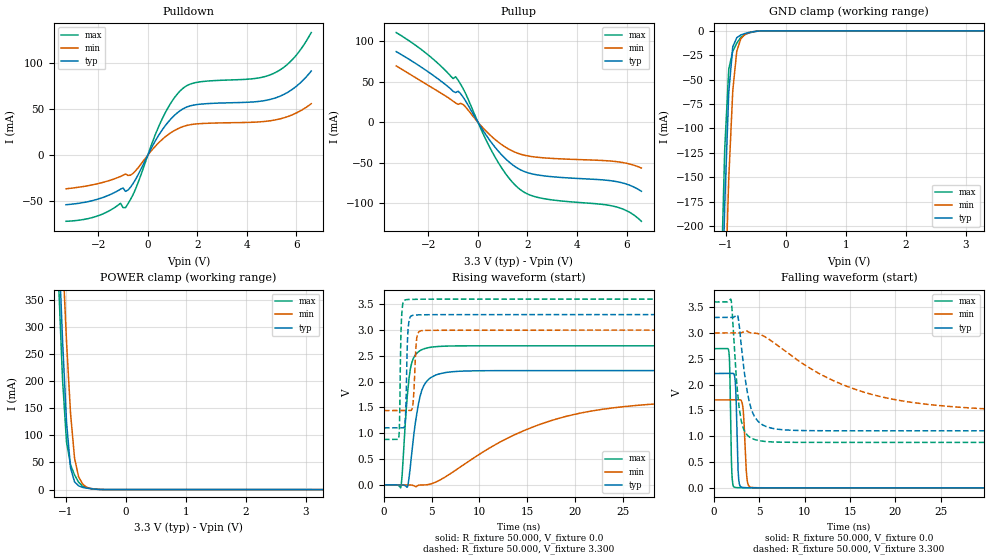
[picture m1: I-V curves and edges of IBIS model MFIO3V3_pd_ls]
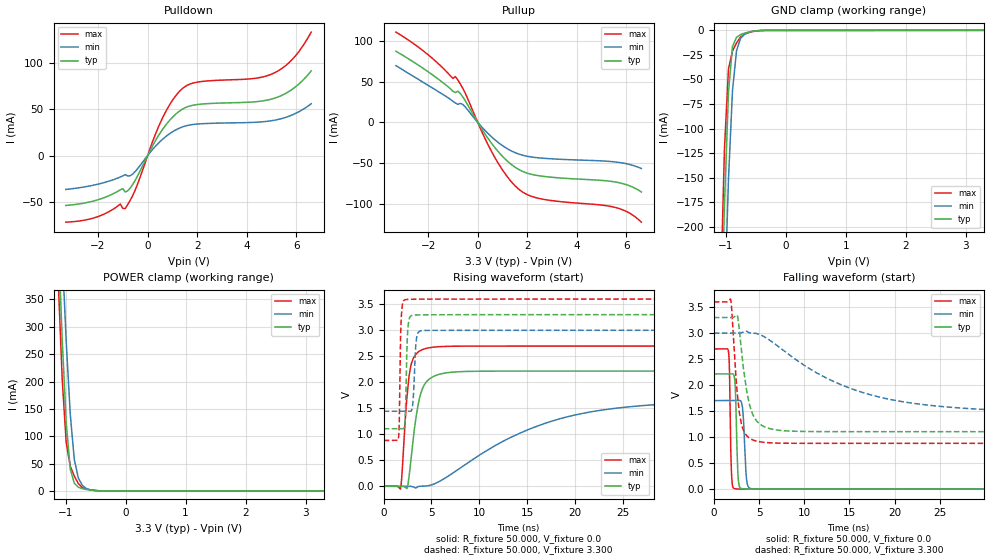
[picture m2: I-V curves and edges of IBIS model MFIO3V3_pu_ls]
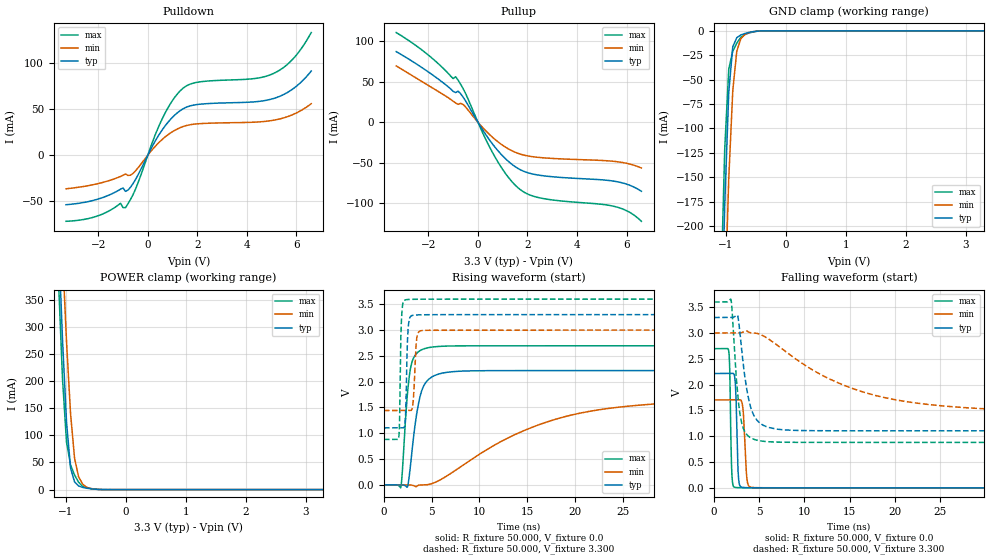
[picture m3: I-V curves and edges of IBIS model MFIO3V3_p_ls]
| IBIS file lpc55s1x_hlqfp100.ibs
[IBIS Ver]   5.0
[File name]   lpc55s1x_hlqfp100.ibs
[File Rev]   1.0
[Date]   June 18,2020
[Notes]   Rev History
|   1.0  initial release
[Disclaimer]   The model given below represents a 100-pin package.
[Copyright]   Copyright NXP 2020
|   Component lpc55s1x:hlqfp100
[Component] lpc55s1x
[Manufacturer] NXP
[Package]
|   typ   min   max
R_pkg   0.19438   0.14402   0.24011
L_pkg   4.719e-9   3.23e-9   5.804e-9
C_pkg   9.634e-13   4.793e-13   1.204e-12
[Pin]   Signal_name   model_name   R_pin   L_pin   C_pin
49   VBAT_DCDC   POWER   NA   NA   NA
50   VBAT_DCDC   POWER   NA   NA   NA
51   VBAT_PMU   POWER   NA   NA   NA
36   USB1_VBUS   POWER   NA   NA   NA
16   VDDA   POWER   NA   NA   NA
38   USB1_3V3   POWER   NA   NA   NA
96   USB0_3V3   POWER   NA   NA   NA
15   VDD   POWER   NA   NA   NA
25   VDD   POWER   NA   NA   NA
44   VDD   POWER   NA   NA   NA
63   VDD   POWER   NA   NA   NA
69   VDD   POWER   NA   NA   NA
75   VDD   POWER   NA   NA   NA
84   VDD   POWER   NA   NA   NA
95   VDD   POWER   NA   NA   NA
100   VDD   POWER   NA   NA   NA
39   VDD_PMU   POWER   NA   NA   NA
18   VREFN   NC   NA   NA   NA
17   VREFP   NC   NA   NA   NA
35   USB1_DM   NC   0.19961   3.9e-9   9.294e-13
34   USB1_DP   NC   0.20574   3.929e-9   9.444e-13
45   FB   NC   0.21411   3.71e-9   9.853e-13
48   LX   NC   0.14402   3.23e-9   1.143e-12
54   P0_0   gpio3v3   0.19671   5.046e-9   1.049e-12
7   P0_1   gpio3v3   0.18569   4.992e-9   9.758e-13
81   P0_2   gpio3v3   0.18955   4.93e-9   9.875e-13
83   P0_3   gpio3v3   0.20167   4.238e-9   9.373e-13
86   P0_4   gpio3v3   0.18453   4.604e-9   8.863e-13
88   P0_5   gpio3v3   0.17208   4.306e-9   4.861e-13
89   P0_6   gpio3v3   0.17688   4.76e-9   7.265e-13
6   P0_7   gpio3v3   0.18495   5.039e-9   9.877e-13
26   P0_8   gpio3v3   0.21082   5.764e-9   9.285e-13
55   P0_9   gpio3v3   0.18836   5.025e-9   1.013e-12
21   P0_10   gpio3v3   0.19767   4.742e-9   1.021e-12
13   P0_11   gpio3v3   0.16852   4.222e-9   4.793e-13
12   P0_12   gpio3v3   0.17445   4.737e-9   7.278e-13
71   P0_13   iicgpio3v3   0.20322   4.784e-9   1.026e-12
72   P0_14   iicgpio3v3   0.2062   5.002e-9   1.056e-12
22   P0_15   gpio3v3   0.20092   4.95e-9   1.063e-12
14   P0_16   gpio3v3   0.19182   3.934e-9   7.286e-13
8   P0_17   gpio3v3   0.18117   4.899e-9   9.571e-13
56   P0_18   gpio3v3   0.18284   4.955e-9   9.928e-13
90   P0_19   gpio3v3   0.17759   4.73e-9   8.974e-13
74   P0_20   gpio3v3   0.24011   4.357e-9   1.204e-12
76   P0_21   gpio3v3   0.21092   5.779e-9   9.242e-13
20   P0_22   gpio3v3   0.20457   4.183e-9   9.919e-13
78   P0_23   gpio3v3   0.19658   5.322e-9   1.084e-12
70   P0_24   gpio3v3   0.21211   4.242e-9   9.876e-13
79   P0_25   gpio3v3   0.19312   5.22e-9   1.048e-12
27   P0_26   gpio3v3   0.197   5.359e-9   1.171e-12
60   P0_27   gpio3v3   0.17389   4.719e-9   9.122e-13
66   P0_28   gpio3v3   0.18341   4.705e-9   9.109e-13
92   P0_29   gpio3v3   0.18226   4.694e-9   9.27e-13
23   P0_30   gpio3v3   0.21051   4.951e-9   1.105e-12
94   P0_31   gpio3v3   0.20907   4.051e-9   9.845e-13
11   P1_0   gpio3v3   0.17643   4.76e-9   9.003e-13
59   P1_1   gpio3v3   0.17508   4.772e-9   9.158e-13
61   P1_2   gpio3v3   0.17391   4.681e-9   9e-13
62   P1_3   gpio3v3   0.17584   4.65e-9   7.307e-13
1   P1_4   gpio3v3   0.21145   5.804e-9   9.228e-13
31   P1_5   gpio3v3   0.1979   4.791e-9   1.002e-12
5   P1_6   gpio3v3   0.19021   5.17e-9   1.023e-12
9   P1_7   gpio3v3   0.17814   4.834e-9   9.098e-13
10   P1_8   gpio3v3   0.1792   4.817e-9   9.052e-13
24   P1_9   gpio3v3   0.22787   4.483e-9   1.184e-12
40   P1_10   gpio3v3   0.19298   4.016e-9   8.906e-13
93   P1_11   gpio3v3   0.19014   4.583e-9   9.519e-13
67   P1_12   gpio3v3   0.19991   4.733e-9   9.253e-13
2   P1_13   gpio3v3   0.19954   5.432e-9   1.175e-12
57   P1_14   gpio3v3   0.17887   4.872e-9   9.721e-13
82   P1_15   gpio3v3   0.1908   4.68e-9   9.803e-13
43   P1_16   gpio3v3   0.20312   4.087e-9   9.402e-13
87   P1_17   gpio3v3   0.18016   4.71e-9   7.274e-13
64   P1_18   gpio3v3   0.17645   4.681e-9   7.229e-13
58   P1_19   gpio3v3   0.1767   4.814e-9   9.428e-13
4   P1_20   gpio3v3   0.19631   5.293e-9   1.056e-12
30   P1_21   gpio3v3   0.19856   5.07e-9   1.02e-12
41   P1_22   gpio3v3   0.18488   4.442e-9   9.08e-13
42   P1_23   gpio3v3   0.18716   4.441e-9   9.092e-13
3   P1_24   gpio3v3   0.20078   5.394e-9   1.079e-12
77   P1_25   gpio3v3   0.19946   5.414e-9   1.191e-12
68   P1_26   gpio3v3   0.20751   4.306e-9   9.447e-13
85   P1_27   gpio3v3   0.19867   4.289e-9   8.839e-13
73   P1_28   gpio3v3   0.21386   4.888e-9   1.092e-12
65   P1_29   gpio3v3   0.17885   4.696e-9   9.052e-13
80   P1_30   gpio3v3   0.18891   5.065e-9   1.012e-12
91   P1_31   gpio3v3   0.17881   4.709e-9   9.248e-13
32   RESETN   gpio3v3   0.2115   4.197e-9   9.778e-13
97   USB0_DP   NC   0.22563   4.185e-9   1.051e-12
98   USB0_DM   NC   0.23166   4.181e-9   1.087e-12
53   XTAL32K_N   NC   0.20814   4.918e-9   1.089e-12
52   XTAL32K_P   NC   0.23349   4.374e-9   1.189e-12
28   XTAL32M_N   NC   0.20639   5.416e-9   1.083e-12
29   XTAL32M_P   NC   0.20019   5.253e-9   1.052e-12
101   VSS   GND   NA   NA   NA
19   VSSA   GND   NA   NA   NA
33   USB1_VSS   GND   NA   NA   NA
37   USB1_VSS   GND   NA   NA   NA
47   VSS_DCDC   GND   NA   NA   NA
46   VSS_DCDC   GND   NA   NA   NA
99   USB0_VSS   GND   NA   NA   NA
|   Model Selector
[Model Selector] gpio3v3
MFIO3V3_pd_hs  EPUN=1 EPD=1 EHS=1
MFIO3V3_pd_ls  EPUN=1 EPD=1 EHS=0
MFIO3V3_pu_hs  EPUN=0 EPD=0 EHS=1
MFIO3V3_pu_ls  EPUN=0 EPD=0 EHS=0
MFIO3V3_p_hs  EPUN=1 EPD=0 EHS=1
MFIO3V3_p_ls  EPUN=1 EPD=0 EHS=0
MFIO3V3_r_hs  EPUN=0 EPD=1 EHS=1
MFIO3V3_r_ls  EPUN=0 EPD=1 EHS=0
[Model Selector] iicgpio3v3
IIC3V3_pd_hs  EGP=1 EPUN=1 EPD=1 EHS=1
IIC3V3_pd_ls  EGP=1 EPUN=1 EPD=1 EHS=0
IIC3V3_p_hs  EGP=1 EPUN=1 EPD=0 EHS=1
IIC3V3_p_ls  EGP=1 EPUN=1 EPD=0 EHS=0
IIC3V3_pu_hs  EGP=1 EPUN=0 EPD=0 EHS=1
IIC3V3_pu_ls  EGP=1 EPUN=0 EPD=0 EHS=0
IIC3V3_r_hs  EGP=1 EPUN=0 EPD=1 EHS=1
IIC3V3_r_ls  EGP=1 EPUN=0 EPD=1 EHS=0
IIC3V3_pd_iic_hs  EGP=0 ECS=0 EPUN=1 EPD=1
IIC3V3_p_iic_hs  EGP=0 ECS=0 EPUN=1 EPD=0
IIC3V3_pu_iic_hs  EGP=0 ECS=0 EPUN=0 EPD=0
IIC3V3_r_iic_hs  EGP=0 ECS=0 EPUN=0 EPD=1
IIC3V3_pd_iic_pu_hs  EGP=0 ECS=1 EPUN=1 EPD=1  SSEL=1
IIC3V3_p_iic_pu_hs  EGP=0 ECS=1 EPUN=1 EPD=0  SSEL=1
IIC3V3_pu_iic_pu_hs  EGP=0 ECS=1 EPUN=0 EPD=0  SSEL=1
IIC3V3_r_iic_pu_hs  EGP=0 ECS=1 EPUN=0 EPD=1  SSEL=1
| Models and submodels in the file (24): MFIO3V3_pd_hs (I/O), MFIO3V3_pd_ls (I/O), MFIO3V3_pu_hs (I/O), MFIO3V3_pu_ls (I/O), MFIO3V3_p_hs (I/O), MFIO3V3_p_ls (I/O), MFIO3V3_r_hs (I/O), MFIO3V3_r_ls (I/O), IIC3V3_pd_hs (I/O), IIC3V3_pd_ls (I/O), IIC3V3_p_hs (I/O), IIC3V3_p_ls (I/O), IIC3V3_pu_hs (I/O), IIC3V3_pu_ls (I/O), IIC3V3_r_hs (I/O), IIC3V3_r_ls (I/O), IIC3V3_pd_iic_hs (I/O_open_drain), IIC3V3_p_iic_hs (I/O_open_drain), IIC3V3_pu_iic_hs (I/O_open_drain), IIC3V3_r_iic_hs (I/O_open_drain), IIC3V3_pd_iic_pu_hs (I/O_open_drain), IIC3V3_p_iic_pu_hs (I/O_open_drain), IIC3V3_pu_iic_pu_hs (I/O_open_drain), IIC3V3_r_iic_pu_hs (I/O_open_drain)
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|   Model MFIO3V3_pd_ls
[Model] MFIO3V3_pd_ls
Model_type I/O
Polarity   Non-Inverting
Enable   Active-Low
Vinl =  0.990V
Vinh =  2.310V
Vmeas =  1.650V
Cref =  0.0F
Rref =  100.000
Vref =  0.0V
C_comp   1.906pF   1.877pF   1.925pF
C_comp_pullup   1.141pF   1.113pF   1.145pF
C_comp_pulldown   0.641pF   0.601pF   0.647pF
[Model Spec]
Vinh   2.310V   2.100V   2.520V
Vinl   0.990V   0.900V   1.080V
Vmeas   1.650V   1.500V   1.800V
Vref   0.0V   0.0V   0.0V
Cref   0.0F   0.0F   0.0F
Rref   100.000   100.000   100.000
[Temperature Range]   25.000   0.125k   -40.000
[Voltage Range]   3.300V   3.000V   3.600V
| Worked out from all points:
|   slope of the pulldown table from 0 to 0.495 V, typ, clamps not added: 20.7 ohm
|   slope of the pullup table from 0 to 0.495 V, typ, clamps not added: 21.4 ohm
|   GND clamp passes 1 mA (typ) near -0.56 V on its own axis
|   POWER clamp passes 1 mA (typ) near -0.53 V on its own axis
|   rising waveform, R_fixture 50.000, V_fixture 0.0: 20-80 % time 1.05ns typ, 11.9ns min, 670ps max; typ from 0 V to 2.21 V
|   rising waveform, R_fixture 50.000, V_fixture 3.300: 20-80 % time 176ps typ, 234ps min, 146ps max; typ from 1.1 V to 3.3 V
|   falling waveform, R_fixture 50.000, V_fixture 0.0: 20-80 % time 203ps typ, 279ps min, 162ps max; typ from 2.21 V to 0 V
|   falling waveform, R_fixture 50.000, V_fixture 3.300: 20-80 % time 1.13ns typ, 11.2ns min, 744ps max; typ from 3.3 V to 1.1 V
[Pulldown]
|Voltage   I(typ)   I(min)   I(max)
-3.3V     -53.7mA    -36.43mA   -71.67mA
-2.1V     -48.29mA   -31.37mA   -66.51mA
-1.1V     -36.82mA   -23.05mA   -52.1mA
-900mV    -39.2mA    -20.39mA   -56.91mA
-600mV    -30.96mA   -19.83mA   -42.97mA
600mV     28.07mA    17.5mA     40.4mA
1V        41.17mA    25.53mA    59.41mA
1.4V      49.87mA    30.79mA    72.04mA
2V        54.93mA    33.94mA    79.03mA
5V        60.84mA    37.53mA    87.68mA
5.9V      72.62mA    44.52mA    105.4mA
6.6V      91.19mA    55.78mA    132.9mA
[Pullup]
|Voltage   I(typ)   I(min)   I(max)
-3.3V     87.16mA    69.54mA    110.7mA
-2.1V     64.12mA    47.22mA    85.31mA
-1V       38.1mA     25.85mA    53.88mA
-900mV    36.64mA    23.75mA    56.16mA
-800mV    38.25mA    22.02mA    51.93mA
-600mV    31.06mA    21.93mA    41.58mA
700mV     -31.25mA   -21.55mA   -43.56mA
1.2V      -47.6mA    -32.42mA   -66.97mA
1.7V      -58.52mA   -39.3mA    -83.05mA
2.6V      -66.01mA   -43.88mA   -94.06mA
5.6V      -73.4mA    -48.74mA   -104.7mA
6.6V      -85.32mA   -56.6mA    -122.4mA
[GND_clamp]
|Voltage   I(typ)   I(min)   I(max)
-3.3V     -7.222A    -7.177A    -7.278A
-1.089V   -337.1mA   -440.8mA   -274.1mA
-1.022V   -178.2mA   -284.2mA   -121mA
-955mV    -63.05mA   -151.6mA   -39.25mA
-888mV    -16.33mA   -61.34mA   -20.9mA
-821mV    -7.066mA   -20.84mA   -12.66mA
-754mV    -4.265mA   -8.157mA   -6.693mA
-687mV    -2.794mA   -3.896mA   -3.841mA
-620mV    -1.725mA   -1.894mA   -2.339mA
-419mV    -112.4uA   -138.2uA   -135uA
3.3V      0A         0A         0A
[POWER_clamp]
|Voltage   I(typ)   I(min)   I(max)
-3.3V     8.016A     7.986A     8.074A
-1.122V   463.8mA    614.4mA    385mA
-1.055V   276.3mA    435mA      203.9mA
-988mV    124.1mA    272.4mA    87.22mA
-921mV    40.03mA    140.2mA    45.68mA
-854mV    14.24mA    57.83mA    27.12mA
-787mV    6.921mA    23.8mA     13.77mA
-720mV    4.141mA    10.27mA    6.207mA
-653mV    2.682mA    4.42mA     3.699mA
-586mV    1.616mA    1.919mA    2.191mA
-452mV    346.9uA    411.9uA    422.9uA
3.3V      0A         0A         0A
[Ramp]
| variable   typ   min   max
dV/dt_r   1.328/1.048n   1.021/11.887n   1.617/0.670n
dV/dt_f   1.317/1.132n   0.935/11.171n   1.631/0.743n
R_load = 50.000
[Rising Waveform]
R_fixture= 50.000
V_fixture= 0.0
V_fixture_min= 0.0
V_fixture_max= 0.0
|time   V(typ)   V(min)   V(max)
0s        11.38nV    124.8nV    46.5nV
1.76ns    11.77uV    -379.4nV   -52.39mV
1.89ns    124.5uV    -254.1nV   156mV
2.47ns    -34.09mV   65.71uV    1.767V
2.93ns    642.6mV    -4.824mV   2.378V
3.75ns    1.693V     -3.224mV   2.598V
4.9ns     2.078V     17.79mV    2.667V
15.38ns   2.214V     1.106V     2.695V
25.84ns   2.214V     1.529V     2.695V
100ns     2.214V     1.702V     2.695V
[Rising Waveform]
R_fixture= 50.000
V_fixture= 3.300
V_fixture_min= 3.000
V_fixture_max= 3.600
|time   V(typ)   V(min)   V(max)
0s        1.105V     1.44V      880.4mV
1.55ns    1.105V     1.44V      919.2mV
1.85ns    1.105V     1.44V      3.271V
2.2ns     1.184V     1.44V      3.582V
2.34ns    1.855V     1.44V      3.589V
2.64ns    3.192V     1.44V      3.594V
3.07ns    3.287V     1.621V     3.596V
3.43ns    3.293V     2.839V     3.597V
4.06ns    3.296V     2.992V     3.598V
100ns     3.299V     2.999V     3.599V
[Falling Waveform]
R_fixture= 50.000
V_fixture= 0.0
V_fixture_min= 0.0
V_fixture_max= 0.0
|time   V(typ)   V(min)   V(max)
0s        2.214V     1.703V     2.695V
1.63ns    2.214V     1.703V     2.64V
1.73ns    2.214V     1.703V     2.3V
1.97ns    2.214V     1.703V     263mV
2.38ns    1.941V     1.702V     7.184mV
2.7ns     199.7mV    1.703V     3.012mV
3.2ns     7.193mV    1.527V     1.541mV
3.63ns    2.938mV    178.8mV    1.008mV
4.26ns    1.462mV    6.421mV    552.8uV
100ns     15.88nV    209.7nV    49.27nV
[Falling Waveform]
R_fixture= 50.000
V_fixture= 3.300
V_fixture_min= 3.000
V_fixture_max= 3.600
|time   V(typ)   V(min)   V(max)
0s        3.299V     2.999V     3.599V
1.87ns    3.299V     2.999V     3.646V
2.6ns     3.336V     2.999V     1.836V
3.1ns     2.603V     3.009V     1.222V
3.85ns    1.693V     3.011V     992.4mV
4.41ns    1.398V     2.998V     939.4mV
5.16ns    1.242V     2.965V     908.2mV
14.39ns   1.105V     1.984V     880.4mV
25.09ns   1.105V     1.589V     880.4mV
100ns     1.105V     1.44V      880.4mV
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|   Model MFIO3V3_pu_ls
[Model] MFIO3V3_pu_ls
Model_type I/O
Polarity   Non-Inverting
Enable   Active-Low
Vinl =  0.990V
Vinh =  2.310V
Vmeas =  1.650V
Cref =  0.0F
Rref =  100.000
Vref =  0.0V
C_comp   1.906pF   1.877pF   1.925pF
C_comp_pullup   1.139pF   1.112pF   1.144pF
C_comp_pulldown   0.643pF   0.602pF   0.649pF
[Model Spec]
Vinh   2.310V   2.100V   2.520V
Vinl   0.990V   0.900V   1.080V
Vmeas   1.650V   1.500V   1.800V
Vref   0.0V   0.0V   0.0V
Cref   0.0F   0.0F   0.0F
Rref   100.000   100.000   100.000
[Temperature Range]   25.000   0.125k   -40.000
[Voltage Range]   3.300V   3.000V   3.600V
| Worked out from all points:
|   slope of the pulldown table from 0 to 0.495 V, typ, clamps not added: 20.7 ohm
|   slope of the pullup table from 0 to 0.495 V, typ, clamps not added: 21.4 ohm
|   GND clamp passes 1 mA (typ) near -0.55 V on its own axis
|   POWER clamp passes 1 mA (typ) near -0.54 V on its own axis
|   rising waveform, R_fixture 50.000, V_fixture 0.0: 20-80 % time 1.05ns typ, 11.9ns min, 674ps max; typ from 0.001 V to 2.21 V
|   rising waveform, R_fixture 50.000, V_fixture 3.300: 20-80 % time 179ps typ, 230ps min, 146ps max; typ from 1.11 V to 3.3 V
|   falling waveform, R_fixture 50.000, V_fixture 0.0: 20-80 % time 203ps typ, 278ps min, 162ps max; typ from 2.21 V to 0.001 V
|   falling waveform, R_fixture 50.000, V_fixture 3.300: 20-80 % time 1.14ns typ, 11.2ns min, 744ps max; typ from 3.3 V to 1.11 V
[Pulldown]
|Voltage   I(typ)   I(min)   I(max)
-3.3V     -53.7mA    -36.43mA   -71.67mA
-2.1V     -48.29mA   -31.37mA   -66.51mA
-1.1V     -36.82mA   -23.05mA   -52.1mA
-900mV    -39.2mA    -20.39mA   -56.91mA
-600mV    -30.96mA   -19.83mA   -42.97mA
600mV     28.07mA    17.5mA     40.4mA
1V        41.17mA    25.53mA    59.41mA
1.4V      49.87mA    30.79mA    72.04mA
2V        54.93mA    33.94mA    79.03mA
5V        60.84mA    37.53mA    87.68mA
5.9V      72.62mA    44.52mA    105.4mA
6.6V      91.19mA    55.78mA    132.9mA
[Pullup]
|Voltage   I(typ)   I(min)   I(max)
-3.3V     87.16mA    69.54mA    110.7mA
-2.1V     64.12mA    47.22mA    85.31mA
-1V       38.1mA     25.85mA    53.88mA
-900mV    36.64mA    23.75mA    56.16mA
-800mV    38.25mA    22.02mA    51.93mA
-600mV    31.06mA    21.93mA    41.58mA
700mV     -31.25mA   -21.55mA   -43.56mA
1.2V      -47.6mA    -32.42mA   -66.97mA
1.7V      -58.52mA   -39.3mA    -83.05mA
2.6V      -66.01mA   -43.88mA   -94.06mA
5.6V      -73.4mA    -48.74mA   -104.7mA
6.6V      -85.32mA   -56.6mA    -122.4mA
[GND_clamp]
|Voltage   I(typ)   I(min)   I(max)
-3.3V     -7.222A    -7.177A    -7.278A
-1.089V   -337.2mA   -440.9mA   -274.2mA
-1.022V   -178.3mA   -284.2mA   -121.1mA
-955mV    -63.12mA   -151.7mA   -39.33mA
-888mV    -16.39mA   -61.39mA   -20.98mA
-821mV    -7.132mA   -20.89mA   -12.74mA
-754mV    -4.331mA   -8.209mA   -6.777mA
-687mV    -2.86mA    -3.948mA   -3.925mA
-620mV    -1.791mA   -1.946mA   -2.423mA
-419mV    -178.1uA   -190.3uA   -219.1uA
3.3V      0A         0A         0A
[POWER_clamp]
|Voltage   I(typ)   I(min)   I(max)
-3.3V     8.016A     7.986A     8.074A
-1.122V   463.7mA    614.3mA    385mA
-1.055V   276.3mA    434.9mA    203.9mA
-988mV    124mA      272.3mA    87.13mA
-921mV    39.96mA    140.1mA    45.6mA
-854mV    14.17mA    57.77mA    27.03mA
-787mV    6.855mA    23.75mA    13.68mA
-720mV    4.075mA    10.22mA    6.123mA
-653mV    2.616mA    4.368mA    3.615mA
-586mV    1.55mA     1.867mA    2.107mA
-452mV    281.1uA    359.9uA    338.7uA
3.3V      0A         0A         0A
[Ramp]
| variable   typ   min   max
dV/dt_r   1.329/1.048n   1.022/11.881n   1.617/0.670n
dV/dt_f   1.316/1.133n   0.935/11.179n   1.631/0.744n
R_load = 50.000
[Rising Waveform]
R_fixture= 50.000
V_fixture= 0.0
V_fixture_min= 0.0
V_fixture_max= 0.0
|time   V(typ)   V(min)   V(max)
0s        869.8uV    949.2uV    842.8uV
1.76ns    883.1uV    948.8uV    -50.04mV
1.91ns    1.009mV    949.1uV    208mV
2.46ns    -36.02mV   1.012mV    1.752V
2.89ns    574.4mV    -2.122mV   2.352V
3.71ns    1.664V     -1.354mV   2.595V
4.93ns    2.083V     22.11mV    2.669V
15.41ns   2.215V     1.111V     2.696V
25.89ns   2.215V     1.532V     2.696V
100ns     2.215V     1.704V     2.696V
[Rising Waveform]
R_fixture= 50.000
V_fixture= 3.300
V_fixture_min= 3.000
V_fixture_max= 3.600
|time   V(typ)   V(min)   V(max)
0s        1.106V     1.442V     881.7mV
1.55ns    1.106V     1.442V     920.7mV
1.83ns    1.106V     1.442V     3.201V
2.2ns     1.19V      1.442V     3.584V
2.36ns    2.014V     1.442V     3.591V
2.67ns    3.219V     1.441V     3.595V
3.05ns    3.288V     1.591V     3.597V
3.47ns    3.295V     2.885V     3.598V
4.05ns    3.297V     2.994V     3.599V
100ns     3.3V       3V         3.6V
[Falling Waveform]
R_fixture= 50.000
V_fixture= 0.0
V_fixture_min= 0.0
V_fixture_max= 0.0
|time   V(typ)   V(min)   V(max)
0s        2.215V     1.704V     2.696V
1.63ns    2.215V     1.704V     2.641V
1.73ns    2.215V     1.704V     2.3V
1.97ns    2.216V     1.704V     265.9mV
2.37ns    1.988V     1.704V     8.752mV
2.68ns    252.6mV    1.704V     4.211mV
3.22ns    8.138mV    1.493V     2.448mV
3.64ns    3.966mV    165.1mV    1.883mV
4.28ns    2.4mV      8.68mV     1.408mV
100ns     869.8uV    949.4uV    842.8uV
[Falling Waveform]
R_fixture= 50.000
V_fixture= 3.300
V_fixture_min= 3.000
V_fixture_max= 3.600
|time   V(typ)   V(min)   V(max)
0s        3.3V       3V         3.6V
1.88ns    3.3V       3V         3.639V
2.61ns    3.334V     3V         1.817V
3.06ns    2.664V     3.008V     1.251V
3.83ns    1.711V     3.015V     996.5mV
4.37ns    1.414V     3.001V     943.5mV
5.06ns    1.258V     2.975V     912.3mV
14.38ns   1.106V     1.987V     881.7mV
25.08ns   1.106V     1.591V     881.7mV
100ns     1.106V     1.442V     881.7mV
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|   Model MFIO3V3_p_ls
[Model] MFIO3V3_p_ls
Model_type I/O
Polarity   Non-Inverting
Enable   Active-Low
Vinl =  0.990V
Vinh =  2.310V
Vmeas =  1.650V
Cref =  0.0F
Rref =  100.000
Vref =  0.0V
C_comp   1.906pF   1.877pF   1.925pF
C_comp_pullup   1.140pF   1.112pF   1.144pF
C_comp_pulldown   0.642pF   0.602pF   0.649pF
[Model Spec]
Vinh   2.310V   2.100V   2.520V
Vinl   0.990V   0.900V   1.080V
Vmeas   1.650V   1.500V   1.800V
Vref   0.0V   0.0V   0.0V
Cref   0.0F   0.0F   0.0F
Rref   100.000   100.000   100.000
[Temperature Range]   25.000   0.125k   -40.000
[Voltage Range]   3.300V   3.000V   3.600V
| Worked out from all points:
|   slope of the pulldown table from 0 to 0.495 V, typ, clamps not added: 20.7 ohm
|   slope of the pullup table from 0 to 0.495 V, typ, clamps not added: 21.4 ohm
|   GND clamp passes 1 mA (typ) near -0.56 V on its own axis
|   POWER clamp passes 1 mA (typ) near -0.54 V on its own axis
|   rising waveform, R_fixture 50.000, V_fixture 0.0: 20-80 % time 1.05ns typ, 11.9ns min, 670ps max; typ from 0 V to 2.21 V
|   rising waveform, R_fixture 50.000, V_fixture 3.300: 20-80 % time 177ps typ, 237ps min, 147ps max; typ from 1.1 V to 3.3 V
|   falling waveform, R_fixture 50.000, V_fixture 0.0: 20-80 % time 203ps typ, 282ps min, 162ps max; typ from 2.21 V to 0 V
|   falling waveform, R_fixture 50.000, V_fixture 3.300: 20-80 % time 1.14ns typ, 11.2ns min, 740ps max; typ from 3.3 V to 1.1 V
[Pulldown]
|Voltage   I(typ)   I(min)   I(max)
-3.3V     -53.7mA    -36.43mA   -71.67mA
-2.1V     -48.29mA   -31.37mA   -66.51mA
-1.1V     -36.82mA   -23.05mA   -52.1mA
-900mV    -39.2mA    -20.39mA   -56.91mA
-600mV    -30.96mA   -19.83mA   -42.97mA
600mV     28.07mA    17.5mA     40.4mA
1V        41.17mA    25.53mA    59.41mA
1.4V      49.87mA    30.79mA    72.04mA
2V        54.93mA    33.94mA    79.03mA
5V        60.84mA    37.53mA    87.68mA
5.9V      72.62mA    44.52mA    105.4mA
6.6V      91.19mA    55.78mA    132.9mA
[Pullup]
|Voltage   I(typ)   I(min)   I(max)
-3.3V     87.16mA    69.54mA    110.7mA
-2.1V     64.12mA    47.22mA    85.31mA
-1V       38.1mA     25.85mA    53.88mA
-900mV    36.64mA    23.75mA    56.16mA
-800mV    38.25mA    22.02mA    51.93mA
-600mV    31.06mA    21.93mA    41.58mA
700mV     -31.25mA   -21.55mA   -43.56mA
1.2V      -47.6mA    -32.42mA   -66.97mA
1.7V      -58.52mA   -39.3mA    -83.05mA
2.6V      -66.01mA   -43.88mA   -94.06mA
5.6V      -73.4mA    -48.74mA   -104.7mA
6.6V      -85.32mA   -56.6mA    -122.4mA
[GND_clamp]
|Voltage   I(typ)   I(min)   I(max)
-3.3V     -7.222A    -7.177A    -7.278A
-1.089V   -337.1mA   -440.8mA   -274.1mA
-1.022V   -178.2mA   -284.2mA   -121mA
-955mV    -63.04mA   -151.6mA   -39.24mA
-888mV    -16.32mA   -61.33mA   -20.89mA
-821mV    -7.057mA   -20.83mA   -12.64mA
-754mV    -4.256mA   -8.15mA    -6.682mA
-687mV    -2.785mA   -3.888mA   -3.83mA
-620mV    -1.717mA   -1.887mA   -2.329mA
-419mV    -104.8uA   -131.8uA   -126uA
3.3V      0A         0A         0A
[POWER_clamp]
|Voltage   I(typ)   I(min)   I(max)
-3.3V     8.016A     7.986A     8.074A
-1.122V   463.7mA    614.3mA    384.9mA
-1.055V   276.2mA    434.9mA    203.8mA
-988mV    124mA      272.3mA    87.12mA
-921mV    39.95mA    140.1mA    45.59mA
-854mV    14.16mA    57.77mA    27.02mA
-787mV    6.846mA    23.74mA    13.67mA
-720mV    4.066mA    10.21mA    6.113mA
-653mV    2.607mA    4.361mA    3.605mA
-586mV    1.542mA    1.86mA     2.097mA
-452mV    273.4uA    353.7uA    329.6uA
3.3V      0A         0A         0A
[Ramp]
| variable   typ   min   max
dV/dt_r   1.329/1.049n   1.022/11.884n   1.618/0.670n
dV/dt_f   1.317/1.134n   0.935/11.178n   1.632/0.744n
R_load = 50.000
[Rising Waveform]
R_fixture= 50.000
V_fixture= 0.0
V_fixture_min= 0.0
V_fixture_max= 0.0
|time   V(typ)   V(min)   V(max)
0s        11.91nV    127.2nV    48.18nV
1.76ns    14.07uV    -353.2nV   -52.48mV
1.9ns     130.3uV    -106.1nV   185.6mV
2.46ns    -38.99mV   62.57uV    1.761V
2.93ns    644.9mV    -4.797mV   2.378V
3.65ns    1.606V     -5.408mV   2.586V
4.94ns    2.084V     20.24mV    2.669V
15.63ns   2.215V     1.125V     2.696V
25.83ns   2.215V     1.53V      2.696V
100ns     2.215V     1.703V     2.696V
[Rising Waveform]
R_fixture= 50.000
V_fixture= 3.300
V_fixture_min= 3.000
V_fixture_max= 3.600
|time   V(typ)   V(min)   V(max)
0s        1.105V     1.441V     880.7mV
1.55ns    1.105V     1.441V     919.6mV
1.84ns    1.105V     1.441V     3.233V
2.22ns    1.224V     1.441V     3.584V
2.37ns    2.139V     1.441V     3.59V
2.68ns    3.224V     1.44V      3.594V
3.06ns    3.287V     1.603V     3.596V
3.45ns    3.294V     2.861V     3.598V
4.07ns    3.297V     2.993V     3.599V
100ns     3.3V       3V         3.6V
[Falling Waveform]
R_fixture= 50.000
V_fixture= 0.0
V_fixture_min= 0.0
V_fixture_max= 0.0
|time   V(typ)   V(min)   V(max)
0s        2.215V     1.703V     2.696V
1.62ns    2.215V     1.703V     2.651V
1.73ns    2.215V     1.703V     2.303V
1.97ns    2.215V     1.703V     265.7mV
2.37ns    1.981V     1.703V     8.251mV
2.69ns    225.2mV    1.704V     3.621mV
3.22ns    7.595mV    1.492V     1.863mV
3.64ns    3.369mV    166.1mV    1.261mV
4.27ns    1.779mV    7.484mV    732uV
100ns     16.41nV    212.2nV    50.94nV
[Falling Waveform]
R_fixture= 50.000
V_fixture= 3.300
V_fixture_min= 3.000
V_fixture_max= 3.600
|time   V(typ)   V(min)   V(max)
0s        3.3V       3V         3.6V
1.88ns    3.3V       3V         3.641V
2.61ns    3.334V     3V         1.821V
3.08ns    2.642V     3.009V     1.24V
3.83ns    1.711V     3.015V     995.8mV
4.38ns    1.41V      3.001V     942.3mV
5.17ns    1.242V     2.968V     908.5mV
14.42ns   1.105V     1.984V     880.8mV
25.12ns   1.105V     1.59V      880.7mV
100ns     1.105V     1.441V     880.7mV
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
